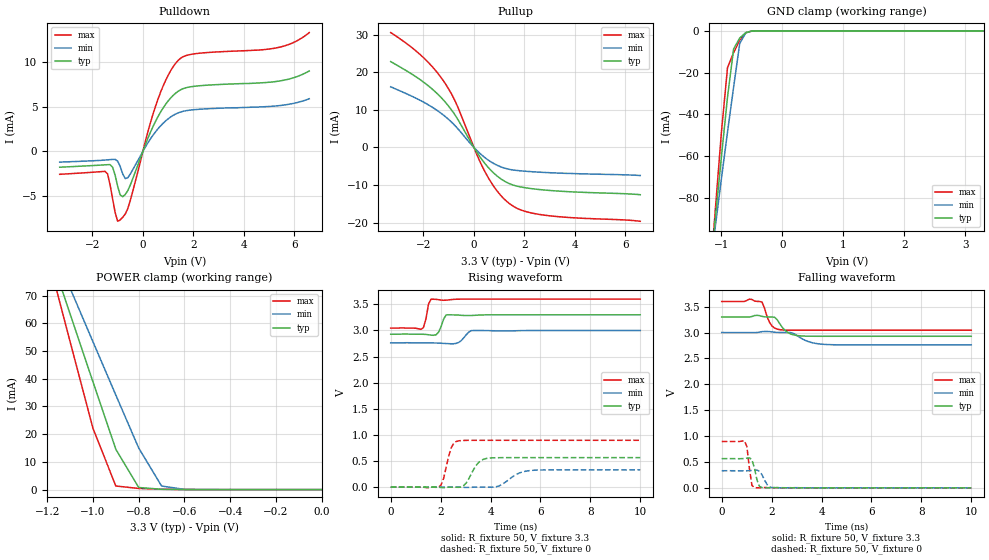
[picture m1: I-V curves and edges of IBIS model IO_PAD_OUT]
[IBIS Ver]   3.2
[Comment Char]   |_char
[File name]   sg-3031cma_33v_.ibs
[File Rev]   1.0
[Date]   2019/10/01 9:58:59
[Source]
[Notes]
[Disclaimer]
This information is for modeling purposes only, and is not guaranteed.
Property of SEIKO EPSON Corp.,
unauthorized reproduction and/or distribution is strictly prohibited.
[Copyright]
Copyright 2019, SEIKO EPSON Corp.
[Component]   G9T010W0A
Si_location Pin
Timing_location Pin
[Manufacturer]   SEIKO EPSON Corp.
| SG-3031CMA
[Package]
R_pkg   0.0m   0.0m   0.0m
L_pkg   0.0n   0.0n   0.0n
C_pkg   0.0p   0.0p   0.0p
[Pin] signal_name   model_name
1   VIO   POWER
2   GND   GND
3   OUT   IO_PAD_OUT
4   Vcc   POWER
| Models and submodels in the file (1): IO_PAD_OUT (3-state)
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[Model]   IO_PAD_OUT
Model_type 3-state
Enable Active-High
Polarity Non-Inverting
Vmeas=1.65
C_comp   2.5p   2.0p   3.0p
[Temperature Range] 25   105   -40
[Voltage Range]   3.3   3.0   3.6
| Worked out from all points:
|   slope of the pulldown table from 0 to 0.495 V, typ, clamps not added: 149 ohm
|   slope of the pullup table from 0 to 0.495 V, typ, clamps not added: 104 ohm
|   GND clamp passes 1 mA (typ) near -0.61 V on its own axis
|   POWER clamp passes 1 mA (typ) near -0.80 V on its own axis
|   falling waveform, R_fixture 50, V_fixture 3.3: 20-80 % time 393ps typ, 606ps min, 273ps max; typ from 3.3 V to 2.93 V
|   falling waveform, R_fixture 50, V_fixture 0: 20-80 % time 177ps typ, 219ps min, 141ps max; typ from 0.565 V to 0 V
|   rising waveform, R_fixture 50, V_fixture 3.3: 20-80 % time 181ps typ, 263ps min, 136ps max; typ from 2.93 V to 3.3 V
|   rising waveform, R_fixture 50, V_fixture 0: 20-80 % time 418ps typ, 623ps min, 275ps max; typ from 0 V to 0.565 V
[Pullup]
-3.3V     22.82mA    16.12mA    30.53mA
-2.1V     17.86mA    12.41mA    24.49mA
-1.6V     15.2mA     10.46mA    21.08mA
-1.2V     12.54mA    8.547mA    17.61mA
-700mV    8.131mA    5.436mA    11.67mA
100mV     -1.093mA   -701.7uA   -1.632mA
500mV     -4.792mA   -3.038mA   -7.214mA
900mV     -7.494mA   -4.673mA   -11.4mA
1.4V      -9.612mA   -5.829mA   -14.9mA
1.9V      -10.57mA   -6.261mA   -16.72mA
2.8V      -11.34mA   -6.663mA   -18.02mA
6.6V      -12.58mA   -7.475mA   -19.65mA
[Pulldown]
-3.3V     -1.756mA   -1.186mA   -2.546mA
-1.5V     -1.492mA   -955.2uA   -2.217mA
-1.4V     -1.474mA   -932uA     -2.501mA
-1.2V     -1.76mA    -888.1uA   -5.292mA
-1V       -3.877mA   -1.074mA   -7.781mA
-900mV    -4.836mA   -1.66mA    -7.626mA
-600mV    -4.375mA   -2.927mA   -6.383mA
500mV     3.345mA    2.178mA    5.018mA
1V        5.617mA    3.63mA     8.471mA
1.4V      6.707mA    4.298mA    10.15mA
5.4V      7.839mA    5.103mA    11.6mA
6.6V      8.97mA     5.873mA    13.24mA
[GND Clamp]
-3.3V     -758.8mA   -621.2mA   -940.1mA
-1.2V     -119.6mA   -117.1mA   -123.7mA
-1.1V     -89.89mA   -93.84mA   -85.78mA
-1V       -60.43mA   -70.87mA   -48.68mA
-900mV    -31.78mA   -48.52mA   -17.64mA
-800mV    -8.711mA   -27.01mA   -10.46mA
-700mV    -3.454mA   -6.089mA   -4.512mA
-600mV    -868.8uA   -934.6uA   -956.3uA
-500mV    -86.23uA   -135.8uA   -52.66uA
-400mV    -4.725uA   -14.7uA    -1.074uA
3.3V      38.26pA    62.15nA    23.1pA
[POWER Clamp]
-3.3V     609.4mA    503mA      751.2mA
-1.2V     87.99mA    92.05mA    84.88mA
-1.1V     63.39mA    72.67mA    53.4mA
-1V       38.88mA    53.35mA    22.1mA
-900mV    14.55mA    34.1mA     1.304mA
-800mV    762uA      14.99mA    407.8uA
-700mV    113uA      1.287mA    132.2uA
-600mV    21.58uA    79.23uA    21.07uA
0V        38.09pA    799.9pA    29pA
[Falling Waveform]
R_fixture=50
V_fixture=3.3
V_fixture_min=3.0
V_fixture_max=3.6
0s        3.3V       3V         3.6V
1.111ns   3.3V       3V         3.646V
1.616ns   3.312V     3.017V     3.587V
1.919ns   3.301V     3.018V     3.194V
2.121ns   3.295V     3.006V     3.087V
2.323ns   3.172V     3.001V     3.056V
2.626ns   3.007V     3.002V     3.046V
3.131ns   2.936V     2.906V     3.045V
4.242ns   2.928V     2.768V     3.045V
10ns      2.928V     2.761V     3.045V
[Falling Waveform]
R_fixture=50
V_fixture=0
V_fixture_min=0
V_fixture_max=0
0s        564.8mV    330.8mV    896.5mV
909.1ps   566.4mV    329.7mV    910.3mV
1.01ns    573.6mV    330.9mV    800.2mV
1.212ns   544.3mV    336.3mV    46.68mV
1.313ns   382.2mV    341.5mV    6.012mV
1.515ns   27.61mV    320.9mV    1.575mV
1.616ns   6.195mV    252.5mV    6.477mV
1.818ns   646.2uV    65.17mV    4.406mV
2.02ns    2.097mV    5.713mV    1.506mV
10ns      0V         0V         0V
[Rising Waveform]
R_fixture=50
V_fixture=3.3
V_fixture_min=3.0
V_fixture_max=3.6
0s        2.928V     2.761V     3.045V
1.313ns   2.927V     2.761V     3.055V
1.414ns   2.924V     2.761V     3.224V
1.515ns   2.918V     2.761V     3.505V
1.616ns   2.911V     2.761V     3.598V
1.919ns   2.969V     2.758V     3.589V
2.222ns   3.297V     2.749V     3.58V
2.727ns   3.294V     2.772V     3.599V
3.232ns   3.287V     2.997V     3.6V
10ns      3.3V       3V         3.6V
[Rising Waveform]
R_fixture=50
V_fixture=0
V_fixture_min=0
V_fixture_max=0
0s        0V         0V         0V
1.919ns   -3.036mV   140.5uV    -1.189mV
2.121ns   -10.15mV   167.7uV    167.2mV
2.424ns   -1.069mV   146.5uV    752.6mV
2.727ns   -3.866mV   -1.466mV   886.7mV
3.03ns    80.94mV    -5.943mV   894.9mV
3.535ns   477.6mV    -682.2uV   896.3mV
3.838ns   548.5mV    -1.993mV   896.5mV
5.556ns   564.7mV    315.6mV    896.5mV
10ns      564.8mV    330.8mV    896.5mV
[Ramp]
R_load=50
dV/dt_r   3.389E-1/4.084E-10   1.985E-1/6.192E-10   5.379E-1/2.663E-10
dV/dt_f   2.233E-1/3.912E-10   1.435E-1/6.015E-10   3.331E-1/2.629E-10
|[End   IO_PAD_OUT
